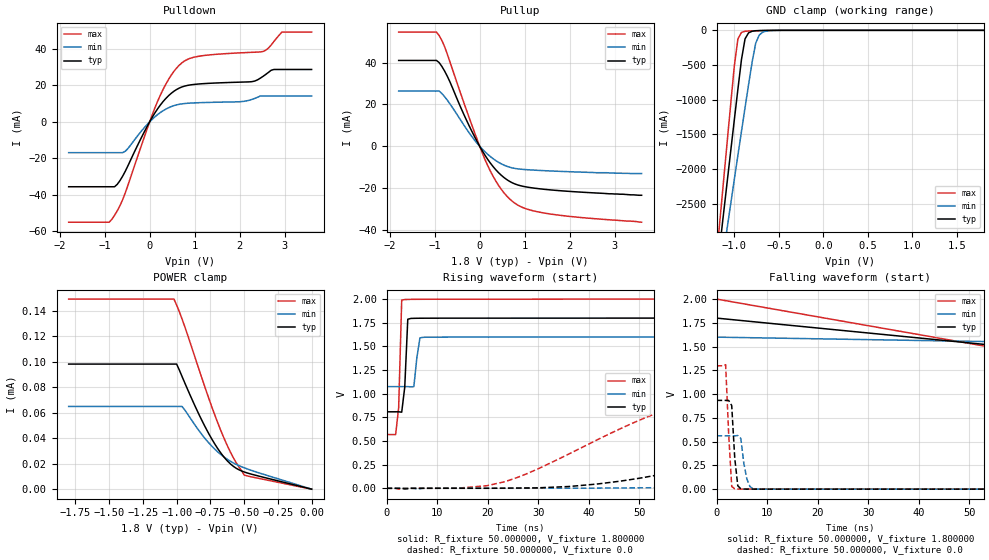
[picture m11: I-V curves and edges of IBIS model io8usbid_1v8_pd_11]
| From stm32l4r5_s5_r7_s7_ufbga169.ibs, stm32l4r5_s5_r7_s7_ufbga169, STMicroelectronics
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|   Model io8usbid_1v8_pd_11
[Model]  io8usbid_1v8_pd_11
Model_type I/O
Polarity   Non-Inverting
Enable   Active-Low
Vinl =   0.540000V
Vinh =   1.260000V
Vmeas =  0.900000V
Cref =   100.000000nF
Rref =   1.000000k
Vref =   1.800000V
C_comp   2.022300pF   2.021100pF   2.049600pF
[Temperature Range]   25.000000   0.125000k   -40.000000
[Pullup Reference]   1.800000V   1.600000V   2.000000V
[Pulldown Reference]   0.0V   0.0V   0.0V
[POWER Clamp Reference]   1.800000V   1.600000V   2.000000V
[GND Clamp Reference]   0.0V   0.0V   0.0V
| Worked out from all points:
|   slope of the pulldown table from 0 to 0.27 V, typ, clamps not added: 26.4 ohm
|   slope of the pullup table from 0 to 0.27 V, typ, clamps not added: 30.1 ohm
|   GND clamp passes 1 mA (typ) near -0.60 V on its own axis
|   rising waveform, R_fixture 50.000000, V_fixture 1.800000: 20-80 % time 587ps typ, 720ps min, 455ps max; typ from 0.808 V to 1.8 V
|   rising waveform, R_fixture 50.000000, V_fixture 0.0: 20-80 % time 65ns typ, 101ns min, 35.5ns max; typ from 0 V to 0.934 V
|   falling waveform, R_fixture 50.000000, V_fixture 1.800000: 20-80 % time 119ns typ, 161ns min, 92ns max; typ from 1.8 V to 0.808 V
|   falling waveform, R_fixture 50.000000, V_fixture 0.0: 20-80 % time 745ps typ, 987ps min, 726ps max; typ from 0.934 V to 0 V
[Pulldown]
|Voltage   I(typ)   I(min)   I(max)
-1.8V     -35.64mA   -16.93mA   -55.1mA
-840mV    -35.64mA   -16.93mA   -53.52mA
-720mV    -34.31mA   -16.93mA   -48.86mA
-540mV    -27.04mA   -16.13mA   -38.89mA
240mV     9.303mA    5.14mA     14.78mA
480mV     15.67mA    8.374mA    25.64mA
720mV     19.18mA    9.883mA    32.46mA
1.14V     20.87mA    10.54mA    36.19mA
2.28V     22.08mA    12.36mA    38.18mA
2.52V     24.96mA    14.19mA    38.63mA
2.94V     28.75mA    14.19mA    49.28mA
3.6V      28.75mA    14.19mA    49.28mA
[Pullup]
|Voltage   I(typ)   I(min)   I(max)
-1.8V     41.08mA    26.4mA     54.65mA
-960mV    41.08mA    26.4mA     54.65mA
-900mV    40.04mA    26.4mA     52.99mA
-780mV    36.03mA    23.75mA    47.71mA
-240mV    10.08mA    6.586mA    14.1mA
120mV     -4.379mA   -2.702mA   -6.45mA
240mV     -8.143mA   -5.004mA   -12mA
420mV     -12.68mA   -7.723mA   -18.77mA
720mV     -17.48mA   -10.36mA   -26.28mA
1.02V     -19.45mA   -11.2mA    -29.88mA
1.5V      -20.78mA   -11.79mA   -32.25mA
3.6V      -23.5mA    -13.1mA    -36.4mA
[GND_clamp]
|Voltage   I(typ)   I(min)   I(max)
-1.8V     -9.895A    -9.296A    -9.457A
-1.2V     -3.533A    -3.902A    -3.274A
-1.16V    -3.082A    -3.55A     -2.716A
-1.12V    -2.631A    -3.198A    -2.159A
-1.08V    -2.182A    -2.848A    -1.604A
-1V       -1.289A    -2.15A     -512mA
-960mV    -849.4mA   -1.803A    -123.8mA
-920mV    -422.4mA   -1.459A    -30.8mA
-880mV    -123.7mA   -1.118A    -13.64mA
-760mV    -6.331mA   -185.1mA   -5.703mA
-680mV    -2.582mA   -25.44mA   -2.917mA
1.8V      47.51uA    51.77uA    39.14uA
[POWER_clamp]
|Voltage   I(typ)   I(min)   I(max)
-1.8V     98.28uA    64.99uA    149.4uA
-1.02V    98.28uA    64.99uA    149.4uA
-1V       98.28uA    64.99uA    144.6uA
-960mV    88.57uA    64.99uA    133.7uA
-820mV    55.53uA    43.9uA     89.47uA
-760mV    43.23uA    36.15uA    70.81uA
-700mV    32.6uA     29.7uA     53.4uA
-640mV    24.05uA    24.57uA    37.82uA
-600mV    19.7uA     21.84uA    28.76uA
-560mV    16.51uA    19.57uA    21uA
-500mV    13.54uA    16.82uA    11.13uA
0V        0A         0A         0A
[Ramp]
| variable   typ   min   max
dV/dt_r  0.56023/65.16690n   0.33674/0.11419u   0.77832/35.46542n
dV/dt_f  0.59462/66.69208n   0.31476/0.11620u   0.85886/35.02316n
R_load = 50.000000
[Rising Waveform]
R_fixture= 50.000000
V_fixture= 1.800000
V_fixture_min= 1.600000
V_fixture_max= 2.000000
|time   V(typ)   V(min)   V(max)
0s        808.4mV    1.075V     568.2mV
1.802ns   808.4mV    1.075V     567.7mV
2.402ns   808.4mV    1.075V     854.7mV
3.003ns   804.6mV    1.075V     1.988V
3.604ns   1.069V     1.075V     1.994V
4.204ns   1.786V     1.075V     1.996V
4.805ns   1.795V     1.072V     1.996V
6.607ns   1.797V     1.589V     1.997V
7.808ns   1.797V     1.597V     1.998V
299.1ns   1.799V     1.599V     2V
[Rising Waveform]
R_fixture= 50.000000
V_fixture= 0.0
V_fixture_min= 0.0
V_fixture_max= 0.0
|time   V(typ)   V(min)   V(max)
0s        166.2uV    292.4uV    105uV
23.42ns   1.801mV    680.9uV    70.23mV
41.44ns   44.38mV    2.261mV    506.4mV
60.06ns   207mV      11.95mV    922.2mV
72.67ns   343.9mV    28.64mV    1.097V
88.89ns   509.5mV    67.29mV    1.211V
119.5ns   730.8mV    178.9mV    1.275V
158ns     864mV      320.9mV    1.293V
219.2ns   922.8mV    480.3mV    1.297V
299.1ns   933.9mV    561.3mV    1.297V
[Falling Waveform]
R_fixture= 50.000000
V_fixture= 1.800000
V_fixture_min= 1.600000
V_fixture_max= 2.000000
|time   V(typ)   V(min)   V(max)
0s        1.799V     1.599V     2V
150.2ns   1.015V     1.468V     597.9mV
300.3ns   821.1mV    1.137V     568.9mV
450.5ns   809.6mV    1.087V     568.2mV
600.6ns   808.4mV    1.077V     568.2mV
900.9ns   808.3mV    1.075V     568.2mV
14.86us   808.4mV    1.075V     568.2mV
[Falling Waveform]
R_fixture= 50.000000
V_fixture= 0.0
V_fixture_min= 0.0
V_fixture_max= 0.0
|time   V(typ)   V(min)   V(max)
0s        933.9mV    561.3mV    1.297V
1.802ns   933.9mV    561.3mV    1.309V
2.402ns   933.1mV    561.3mV    579.6mV
3.003ns   880mV      561.3mV    28.79mV
3.604ns   326.5mV    560.8mV    3.379mV
4.204ns   35.9mV     564.3mV    1.296mV
4.805ns   4.242mV    533.4mV    857.6uV
6.006ns   743.4uV    106.4mV    702.1uV
7.808ns   510.7uV    1.84mV     662.1uV
299.1ns   166.2uV    292.4uV    105uV
